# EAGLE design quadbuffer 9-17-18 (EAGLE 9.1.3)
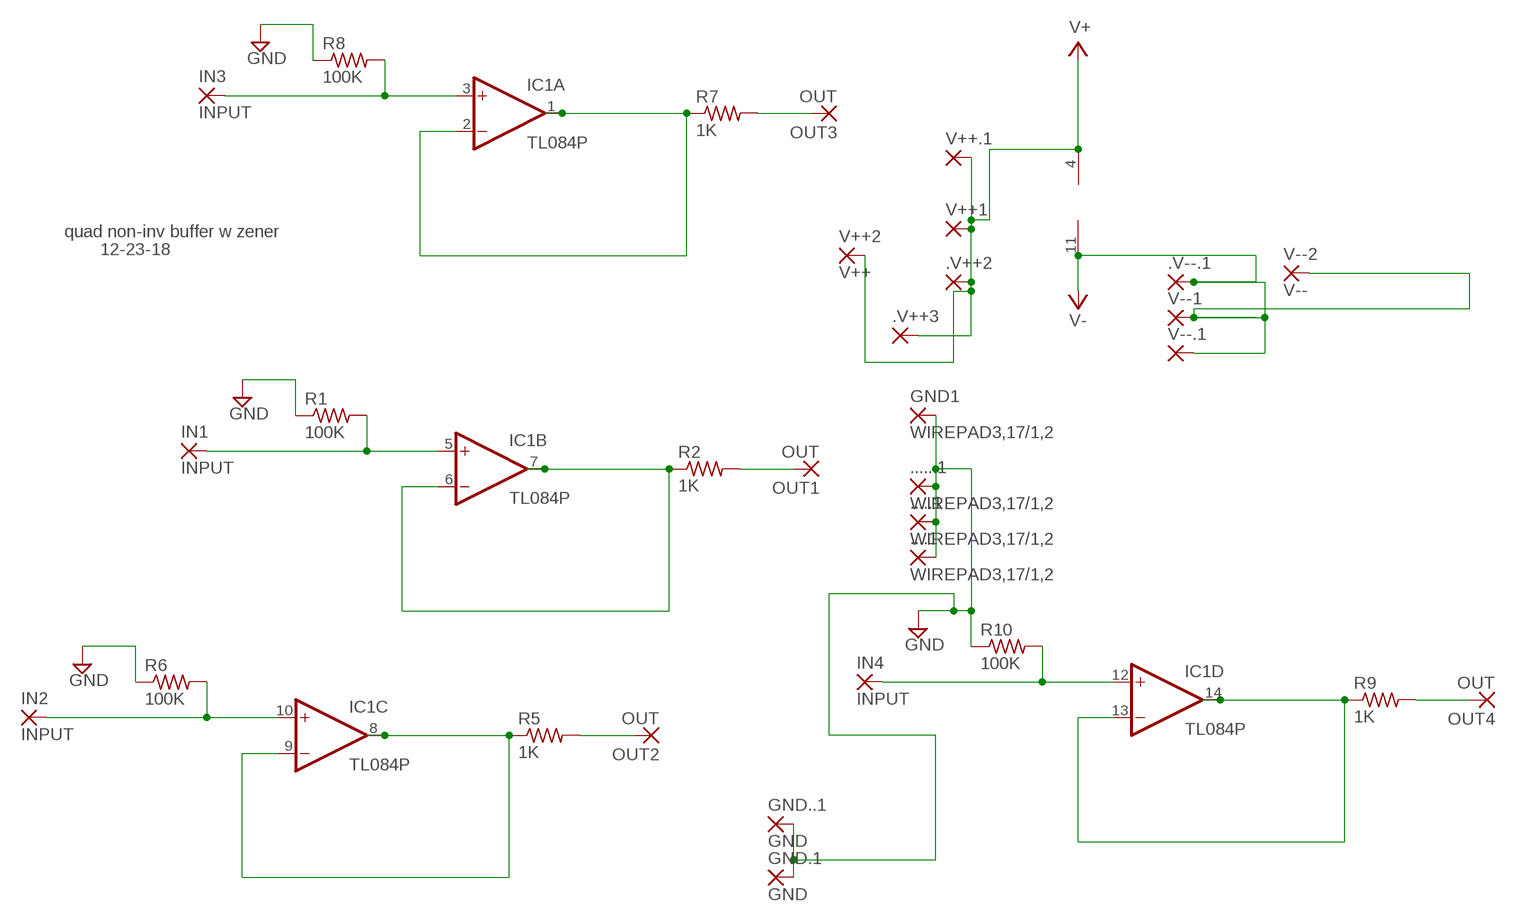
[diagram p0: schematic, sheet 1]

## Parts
....1  WIREPAD3,17/1,2  [3,17/1,2]
.....1  WIREPAD3,17/1,2  [3,17/1,2]
......1  WIREPAD3,17/1,2  [3,17/1,2]
.V++2  2,54/1,0  [2,54/1,0]
.V++3  2,54/1,0  [2,54/1,0]
.V--.1  3,17/1,3  [3,17/1,3]
GND1  WIREPAD3,17/1,2  [3,17/1,2]
GND.1  GND  1,6/0,8  [1,6/0,8]
GND..1  GND  1,6/0,8  [1,6/0,8]
IC1  TL084P  [DIL14]
IN1  INPUT  3,17/1,3  [3,17/1,3]
IN2  INPUT  3,17/1,3  [3,17/1,3]
IN3  INPUT  3,17/1,3  [3,17/1,3]
IN4  INPUT  3,17/1,3  [3,17/1,3]
OUT1  OUT  3,17/1,3  [3,17/1,3]
OUT2  OUT  3,17/1,3  [3,17/1,3]
OUT3  OUT  3,17/1,3  [3,17/1,3]
OUT4  OUT  3,17/1,3  [3,17/1,3]
R1  100K  R-US_0204/7  [0204/7]
R2  1K  R-US_0204/7  [0204/7]
R5  1K  R-US_0204/7  [0204/7]
R6  100K  R-US_0204/7  [0204/7]
R7  1K  R-US_0204/7  [0204/7]
R8  100K  R-US_0204/7  [0204/7]
R9  1K  R-US_0204/7  [0204/7]
R10  100K  R-US_0204/7  [0204/7]
V++1  2,54/1,0  [2,54/1,0]
V++2  V++  1,6/0,8  [1,6/0,8]
V++.1  2,54/1,0  [2,54/1,0]
V--1  3,17/1,3  [3,17/1,3]
V--2  V--  1,6/0,8  [1,6/0,8]
V--.1  3,17/1,3  [3,17/1,3]

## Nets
GND: ....1.1(P) .....1.1(P) ......1.1(P) GND1.1(P) GND.1.1(P) GND..1.1(P) R1.1 R6.1 R8.1 R10.1
N$1: IC1.5(B:+IN) IN1.1(P) R1.2
N$5: OUT2.1(P) R5.2
N$6: IC1.8(C:OUT) IC1.9(C:-IN) R5.1
N$7: IC1.10(C:+IN) IN2.1(P) R6.2
N$8: OUT3.1(P) R7.2
N$9: IC1.1(A:OUT) IC1.2(A:-IN) R7.1
N$10: IC1.3(A:+IN) IN3.1(P) R8.2
N$11: OUT4.1(P) R9.2
N$12: IC1.13(D:-IN) IC1.14(D:OUT) R9.1
N$13: IC1.12(D:+IN) IN4.1(P) R10.2
N$18: IC1.6(B:-IN) IC1.7(B:OUT) R2.1
N$19: OUT1.1(P) R2.2
V+: .V++2.1(P) .V++3.1(P) IC1.4(P:V+) V++1.1(P) V++2.1(P) V++.1.1(P)
V-: .V--.1.1(P) IC1.11(P:V-) V--1.1(P) V--2.1(P) V--.1.1(P)

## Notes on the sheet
- quad non-inv buffer w zener
- 12-23-18

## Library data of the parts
....1 .....1 ......1 GND1 = wirepad-NONAMES:WIREPAD: Wire PAD connect wire on PCB
.V++2 .V++3 V++1 V++.1 = wirepad-NONAMES:2,54/1,0: THROUGH-HOLE PAD
.V--.1 V--1 V--.1 = wirepad-NONAMES:3,17/1,3: THROUGH-HOLE PAD
GND.1 GND..1 V++2 V--2 = wirepad-NONAMES:1,6/0,8: THROUGH-HOLE PAD
IC1 = linear:TL084: OP AMP
IN1-IN4 OUT1-OUT4 = wirepad:3,17/1,3: THROUGH-HOLE PAD
R1 R2 R5-R10 = rcl:R-US_: RESISTOR, American symbol

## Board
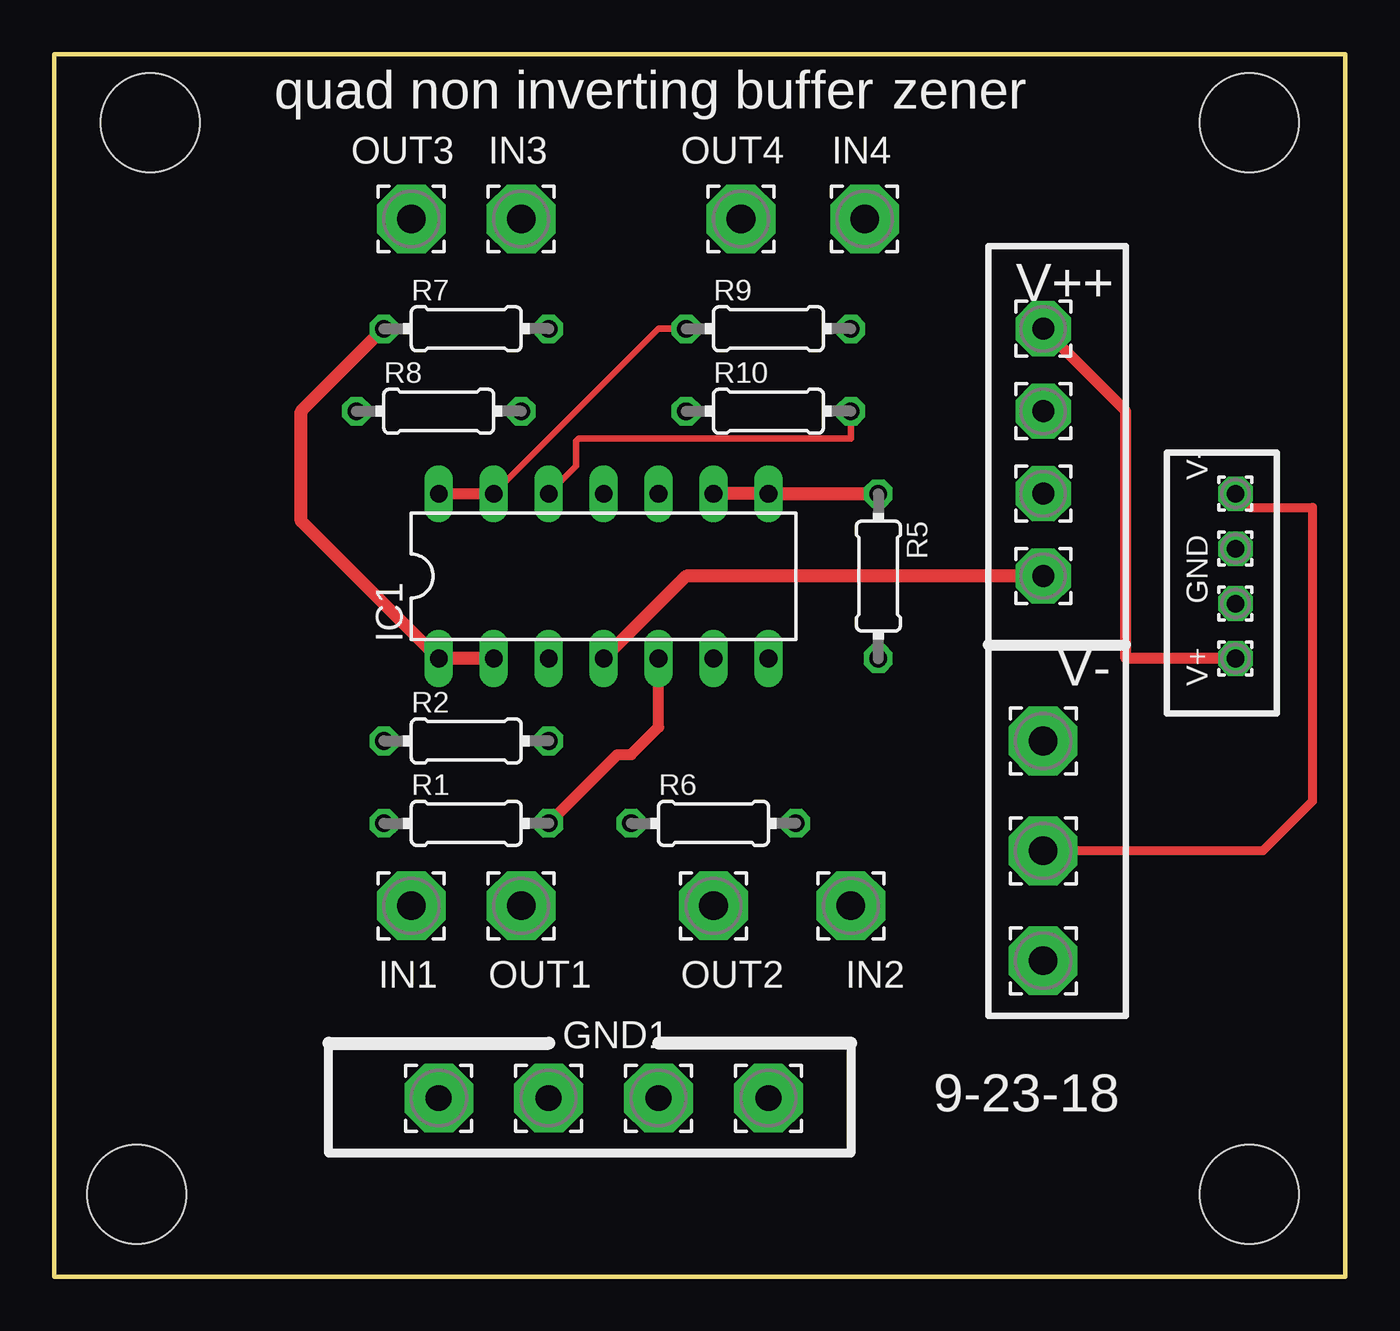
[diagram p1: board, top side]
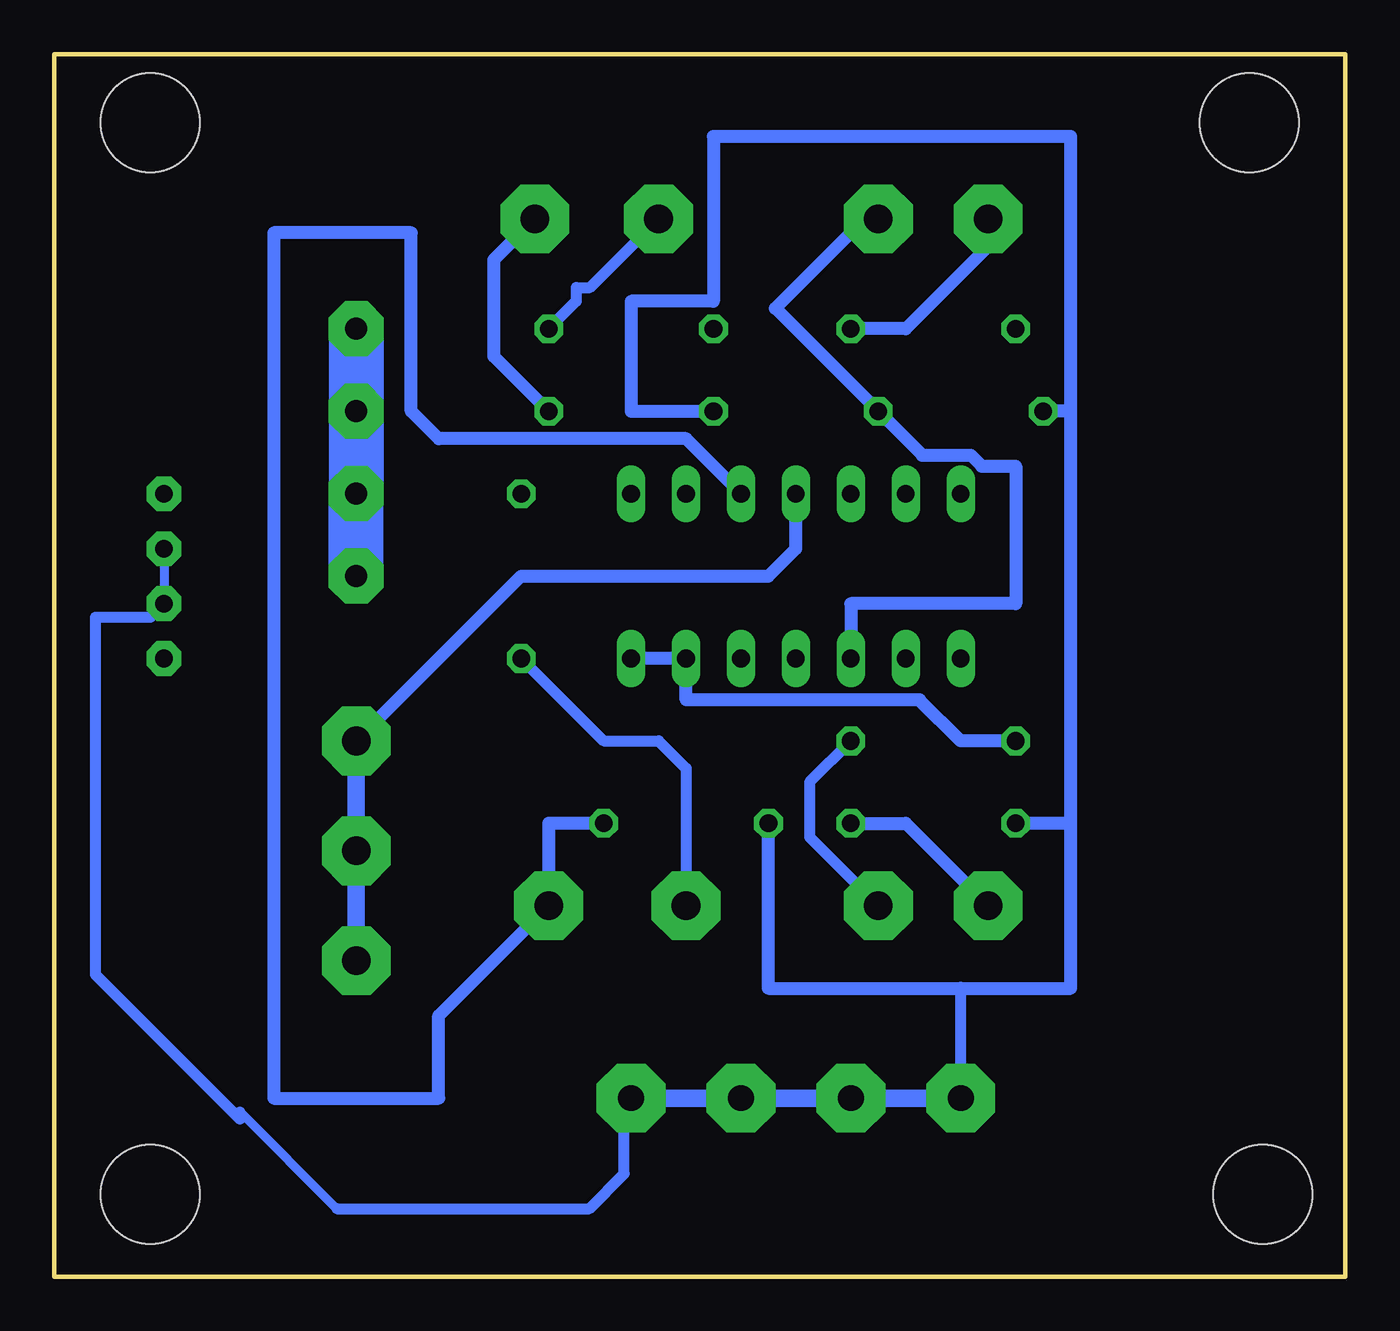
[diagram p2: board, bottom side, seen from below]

Size 59.69 x 56.52 mm. Coordinates in mm from the lower left corner, seen from the top.
Outline: 0,56.52 0,0 59.69,0 59.69,56.52 0,56.52
Copper layers (1*16): Top 0.035mm / dielectric 1.5mm / Bottom 0.035mm
Design rules "default": minimum track width 6mil, minimum drill 0.35mm, track to track 6mil, track to pad 6mil, pad to pad 6mil, via to via 6mil, smd to smd 6mil, copper to edge 40mil, drill to drill 6mil, minimum pad ring 10mil, minimum via ring 8mil, stop-mask expansion 4mil, vias tented up to drill 0mil, thermal gap 10mil
Holes 4.57 mm at 55.24,53.34 3.81,3.81 4.45,53.34 55.24,3.81

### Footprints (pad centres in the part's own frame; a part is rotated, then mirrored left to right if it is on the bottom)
3,17/1,2 = drill 1.194 pad 3.175 octagon: 1 0,0
2,54/1,0 = drill 1.016 pad 2.54 octagon: 1 0,0
3,17/1,3 = drill 1.321 pad 3.175 octagon: 1 0,0
1,6/0,8 = drill 0.813 pad 1.6 octagon: 1 0,0
DIL14 = drill 0.813 long: 1 -7.62,-3.81; 2 -5.08,-3.81; 3 -2.54,-3.81; 4 0,-3.81; 5 2.54,-3.81; 6 5.08,-3.81; 7 7.62,-3.81; 8 7.62,3.81; 9 5.08,3.81; 10 2.54,3.81; 11 0,3.81; 12 -2.54,3.81; 13 -5.08,3.81; 14 -7.62,3.81
0204/7 = drill 0.813 octagon: 1 -3.81,0; 2 3.81,0

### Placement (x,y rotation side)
....1  33.02,8.26 90 top
.....1  27.94,8.26 90 top
......1  22.86,8.26 90 top
.V++2  45.72,40 0 top
.V++3  45.72,32.38 0 top
.V--.1  45.72,14.61 0 top
GND1  17.78,8.26 90 top
GND.1  54.61,33.66 90 top
GND..1  54.61,31.12 90 top
IC1  25.4,32.38 0 top
IN1  16.51,17.14 0 top
IN2  36.83,17.14 0 top
IN3  21.59,48.89 0 top
IN4  37.46,48.89 0 top
OUT1  21.59,17.14 0 top
OUT2  30.48,17.14 0 top
OUT3  16.51,48.89 0 top
OUT4  31.75,48.89 0 top
R1  19.05,20.95 0 top
R2  19.05,24.77 0 top
R5  38.1,32.38 270 top
R6  30.48,20.95 0 top
R7  19.05,43.81 0 top
R8  17.78,40 0 top
R9  33.02,43.81 0 top
R10  33.02,40 0 top
V++1  45.72,43.81 0 top
V++2  54.61,28.57 90 top
V++.1  45.72,36.2 0 top
V--1  45.72,19.68 0 top
V--2  54.61,36.2 90 top
V--.1  45.72,24.77 0 top

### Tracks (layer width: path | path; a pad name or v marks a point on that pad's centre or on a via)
GND
  Bottom 0.406: GND.1.1 GND..1.1 55.24,30.48 | 51.1,7.62 46.63,3.15
  Bottom 0.508: 55.24,30.48 57.78,30.48 57.78,13.97 51.1,7.28 51.1,7.62 | 46.63,3.15 34.95,3.15 33.34,4.76 33.34,7.94 ....1.1 | GND1.1 17.78,13.34
  Bottom 0.61: R6.1 26.67,13.34 17.78,13.34 12.7,13.34 12.7,20.95 | 12.7,20.95 R1.1 | 12.7,20.95 12.7,40 | 12.7,40 R8.1 | 12.7,40 12.7,52.7 29.21,52.7 29.21,45.09 33.02,45.09 33.02,40 R10.1
  Bottom 0.813: ....1.1 .....1.1 ......1.1 GND1.1
N$1
  Top 0.508: R1.2 26.03,24.13 26.67,24.13 27.94,25.4 IC1.5
  Bottom 0.61: R1.2 20.32,20.95 IN1.1
N$5
  Bottom 0.508: R5.2 34.29,24.77 31.75,24.77 30.48,23.49 OUT2.1
N$6
  Top 0.61: R5.1 IC1.8 IC1.9
N$7
  Bottom 0.61: R6.2 36.83,20.95 IN2.1 41.91,12.07 41.91,8.26 49.53,8.26 49.53,48.26 43.18,48.26 43.18,40 41.91,38.73 30.48,38.73 IC1.10
N$8
  Bottom 0.61: OUT3.1 16.51,47.62 20.32,43.81 R7.2
N$9
  Top 0.61: IC1.2 IC1.1 11.43,34.92 11.43,40 R7.1
N$10
  Bottom 0.61: IC1.3 22.86,31.12 15.24,31.12 15.24,37.46 16.81,37.46 17.32,37.97 19.56,37.97 R8.2 26.35,44.77 22.23,48.89 IN3.1
N$11
  Bottom 0.508: OUT4.1 34.92,45.72 35.56,45.72 35.56,45.09 R9.2
N$12
  Top 0.305: IC1.13 27.94,43.81 R9.1
  Top 0.508: IC1.14 IC1.13
N$13
  Top 0.305: IC1.12 24.13,37.46 24.13,38.62 24.25,38.73 36.83,38.73 R10.2
  Bottom 0.61: IN4.1 39.37,46.99 39.37,42.55 R10.2
N$18
  Bottom 0.61: IC1.7 IC1.6 30.48,26.67 19.69,26.67 17.78,24.77 R2.1
N$19
  Bottom 0.508: R2.2 24.77,22.86 24.77,20.32 OUT1.1
V+
  Top 0.508: V++1.1 49.53,40 49.53,28.6 54.59,28.6 V++2.1
  Top 0.61: .V++3.1 29.21,32.38 IC1.4
  Bottom 2.54: V++1.1 .V++2.1 V++.1.1 .V++3.1
V-
  Top 0.406: V--2.1 55.24,35.56 58.17,35.56 58.17,21.97 55.88,19.68 V--1.1
  Bottom 0.61: V--.1.1 38.1,32.38 26.67,32.38 25.4,33.66 IC1.11
  Bottom 0.813: V--.1.1 V--1.1 .V--.1.1

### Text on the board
tNames: quad non inverting buffer | zener | V++ | V- | GND | V- | V+ | 9-23-18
